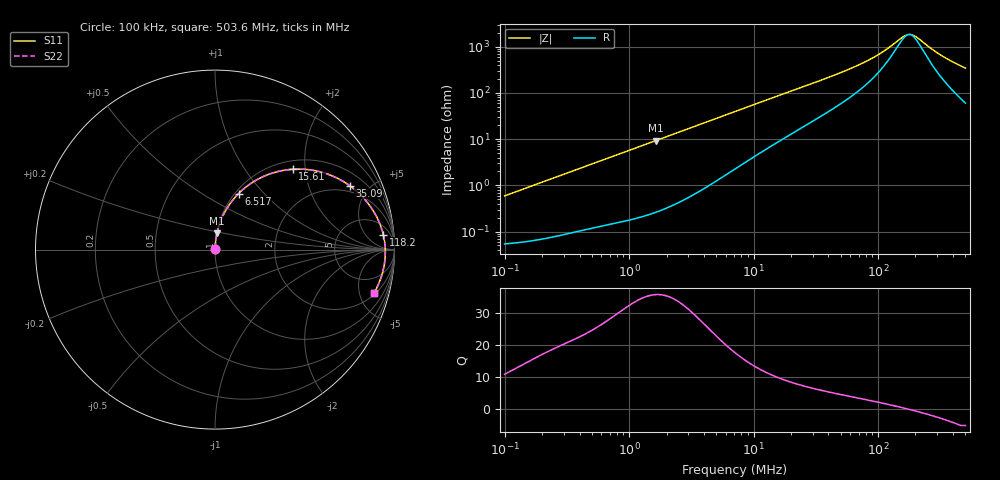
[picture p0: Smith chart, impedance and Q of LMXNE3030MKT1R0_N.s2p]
! LMXNE3030MKT1R0_N  S-PARAMETER MODEL  ( General Type )
! Model Generated by TAIYO YUDEN Corporation (https://www.yuden.co.jp/en/)
! Version 1.0
! TAIYO YUDEN Control No. 191023NI43SB-FBB
! Copyright(c) 2019 TAIYO YUDEN CO.,LTD. All Rights Reserved.
! Product Description (link to TY-COMPAS)
! https://ds.yuden.co.jp/TYCOMPAS/or/detail?pn=LMXNE3030MKT1R0NN&u=M
! Products Name : Inductors
! Characteristics :
!  Inductance : 1.0 uH , SRF(min) : 111 MHz , DC Resistance(max) : 0.0576 Ohm
!  Rated Current : Saturation :2200 mA , Temp Rise : 1710 mA (40 degC)
!  Case Size : 3.0 x 3.0 / 0.118 x 0.118 [mm/inch] , Thickness : 1.2 / 0.047 [mm/inch]
!  (Conditions: Temperature = 25 degC , DC Bias Current/Voltage = 0A / 0V)
! External Node Assignments :
!  1  o---GGG---o  2
! GND o---------o GND
! Frequency Range : 0.1MHz  -  503.601575MHz  [ 402 STEP ]
# MHz S RI R 50
! Freq[MHz].  S11 Real  S11 Imag  S21 Real  S21 Imag  S12 Real  S12 Imag  S22 Real  S22 Imag
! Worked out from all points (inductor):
!   401 points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, 100 kHz to 503.6 MHz, reference 50 ohm
!   read as one part in series: L = 937 nH near 104.4 kHz
!   highest Q = 35.7 at 1.631 MHz (marker M1), where L = 904 nH
!   self-resonance near 177.9 MHz
!   S11 on the Smith chart (normalised r, x): 100 kHz: 1.00, +0.01; 6.517 MHz: 1.04, +0.73; 15.61 MHz: 1.17, +1.71; 35.09 MHz: 1.63, +3.76; 118.2 MHz: 10, +15; 503.6 MHz: 2.21, -6.81
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0.1  0.000573 0.00589  0.9994 -0.00589  0.9994 -0.00589  0.000573 0.00589
0.416965  0.00163 0.0241  0.9984 -0.0241  0.9984 -0.0241  0.00163 0.0241
1.630923  0.011 0.0914  0.989 -0.0914  0.989 -0.0914  0.011 0.0914
1.738598  0.0123 0.0972  0.9877 -0.0972  0.9877 -0.0972  0.0123 0.0972
3.744441  0.0495 0.1997  0.9505 -0.1997  0.9505 -0.1997  0.0495 0.1997
6.516624  0.1312 0.3121  0.8688 -0.3121  0.8688 -0.3121  0.1312 0.3121
7.249345  0.1561 0.3353  0.8439 -0.3353  0.8439 -0.3353  0.1561 0.3353
10.41448  0.2675 0.4064  0.7325 -0.4064  0.7325 -0.4064  0.2675 0.4064
15.61301  0.4323 0.4477  0.5677 -0.4477  0.5677 -0.4477  0.4323 0.4477
21.04067  0.562 0.4389  0.438 -0.4389  0.438 -0.4389  0.562 0.4389
29.58987  0.6945 0.3911  0.3055 -0.3911  0.3055 -0.3911  0.6945 0.3911
35.09012  0.7496 0.3569  0.2504 -0.3569  0.2504 -0.3569  0.7496 0.3569
70.8936  0.894 0.1952  0.106 -0.1952  0.106 -0.1952  0.894 0.1952
93.52439  0.9223 0.1337  0.0777 -0.1337  0.0777 -0.1337  0.9223 0.1337
118.2312  0.9375 0.084  0.0625 -0.084  0.0625 -0.084  0.9375 0.084
123.3794  0.9395 0.0751  0.0605 -0.0751  0.0605 -0.0751  0.9395 0.0751
162.7648  0.9478 0.0182  0.0522 -0.0182  0.0522 -0.0182  0.9478 0.0182
184.966  0.9489 -0.00804  0.0511 0.00804  0.0511 0.00804  0.9489 -0.00804
205.7633  0.9486 -0.0301  0.0514 0.0301  0.0514 0.0301  0.9486 -0.0301
271.4475  0.9422 -0.0894  0.0578 0.0894  0.0578 0.0894  0.9422 -0.0894
328.8386  0.9322 -0.1331  0.0678 0.1331  0.0678 0.1331  0.9322 -0.1331
503.6016  0.8867 -0.2404  0.1133 0.2404  0.1133 0.2404  0.8867 -0.2404
